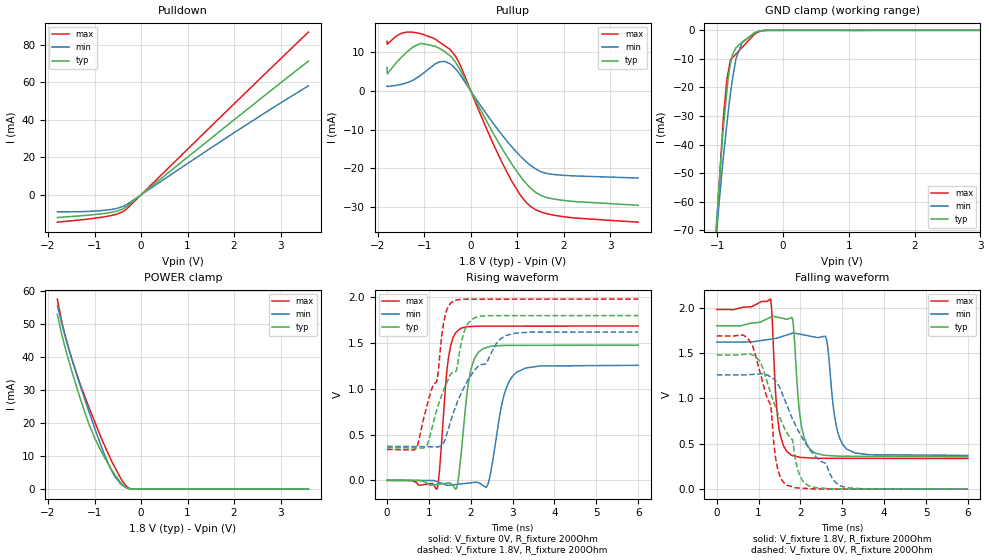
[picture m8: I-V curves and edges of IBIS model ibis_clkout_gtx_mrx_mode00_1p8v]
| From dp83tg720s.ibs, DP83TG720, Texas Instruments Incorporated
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| ibis_clkout_gtx_mrx_mode00_1p8v
[Model]   ibis_clkout_gtx_mrx_mode00_1p8v
Model_type   I/O
Polarity   Non-Inverting
Enable   Active-Low
Vinl = 0.54
Vinh = 1.26
Vmeas = 0.9
Vref = 0.9
Cref = 2pF
Rref = 100000
|   typ   min   max
C_comp   2.97pF   2.96pF   3.01pF
[Voltage Range]   1.8   1.62   1.98
[Temperature Range]   27   150   -40
[Pullup Reference]   1.8   1.62   1.98
[Pulldown Reference]   0   0   0
[Power Clamp Reference]   1.8   1.62   1.98
[GND Clamp Reference]   0   0   0
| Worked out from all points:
|   slope of the pulldown table from 0 to 0.27 V, typ, clamps not added: 49.7 ohm
|   slope of the pullup table from 0 to 0.27 V, typ, clamps not added: 43.2 ohm
|   GND clamp passes 1 mA (typ) near -0.44 V on its own axis
|   POWER clamp passes 1 mA (typ) near -0.37 V on its own axis
|   falling waveform, V_fixture 1.8V, R_fixture 200Ohm: 20-80 % time 172ps typ, 203ps min, 145ps max; typ from 1.8 V to 0.359 V
|   rising waveform, V_fixture 0V, R_fixture 200Ohm: 20-80 % time 219ps typ, 309ps min, 179ps max; typ from 0 V to 1.48 V
|   rising waveform, V_fixture 1.8V, R_fixture 200Ohm: 20-80 % time 662ps typ, 965ps min, 459ps max; typ from 0.359 V to 1.8 V
|   falling waveform, V_fixture 0V, R_fixture 200Ohm: 20-80 % time 691ps typ, 1.03ns min, 411ps max; typ from 1.48 V to 0 V
[Pulldown]
|   Voltage   I(typ)   I(min)   I(max)
-1.8V     -12.08mA   -9.033mA   -14.56mA
-1.125V   -10.8mA    -8.807mA   -12.86mA
-730.8mV  -9.674mA   -8.07mA    -11.45mA
-520.2mV  -8.646mA   -7.206mA   -10.24mA
-336.6mV  -6.645mA   -5.499mA   -8.007mA
2.072V    41.36mA    34.22mA    50.17mA
3.6V      71.25mA    58.08mA    86.69mA
[GND Clamp]
|   Voltage   I(typ)   I(min)   I(max)
-1.8V     -382.3mA   -332mA     -425.2mA
-1.017V   -68.67mA   -71.81mA   -70.53mA
-903.6mV  -32.69mA   -43.18mA   -29.12mA
-855mV    -21.28mA   -32.69mA   -17.07mA
-838.8mV  -17.47mA   -29.2mA    -15.06mA
-801mV    -11.68mA   -22.1mA    -10.37mA
-774mV    -8.705mA   -17.42mA   -9.699mA
-714.6mV  -6.046mA   -9.737mA   -8.229mA
-622.8mV  -4.089mA   -4.277mA   -5.956mA
-444.6mV  -1.097mA   -993.2uA   -1.545mA
-261mV    -16.1uA    -40.43uA   -15.49uA
3.6V      0A         0A         0A
[Pullup]
|   Voltage   I(typ)   I(min)   I(max)
-1.8V     6.066mA    1.271mA    12.85mA
-1.789V   4.411mA    1.14mA     12.09mA
-1.476V   8.918mA    1.762mA    15mA
-1.071V   12.31mA    4.113mA    14.83mA
-676.8mV  11.06mA    7.524mA    12.68mA
-444.6mV  9.086mA    7.025mA    10.74mA
-239.4mV  5.662mA    4.354mA    7.043mA
343.8mV   -7.902mA   -6.066mA   -9.904mA
797.4mV   -17.36mA   -13.27mA   -21.5mA
1.278V    -25.1mA    -19.23mA   -29.86mA
1.845V    -28.13mA   -21.74mA   -32.33mA
3.6V      -29.64mA   -22.58mA   -34.02mA
[POWER Clamp]
|   Voltage   I(typ)   I(min)   I(max)
-1.8V     53.01mA    55.74mA    57.65mA
-1.681V   45.61mA    49.02mA    49.43mA
-1.546V   38.55mA    42.1mA     42.27mA
-1.319V   27.98mA    31.92mA    32.33mA
-1.114V   19.49mA    23.28mA    24.54mA
-973.8mV  14.8mA     17.58mA    19.66mA
-666mV    6.684mA    6.531mA    9.544mA
-558mV    4.288mA    3.744mA    6.479mA
-444.6mV  2.137mA    1.736mA    3.468mA
-293.4mV  327.2uA    317.2uA    675uA
-109.8mV  6.037uA    13.6uA     2.646uA
3.6V      0A         0A         0A
[Ramp]
R_load = 200
|   typ   min   max
dV/dt_r   0.886179/2.19298e-10   0.754021/3.07889e-10   1.01172/1.7845e-10
dV/dt_f   0.864917/1.69904e-10   0.748861/2.02115e-10   0.985494/1.43915e-10
[Falling Waveform]
V_fixture = 1.8V
V_fixture_min = 1.62V
V_fixture_max = 1.98V
R_fixture = 200Ohm
C_fixture = 0F
|   Time   V(typ)   V(min)   V(max)
0s        1.8V       1.62V      1.98V
1.282ns   1.893V     1.652V     2.094V
1.469ns   1.892V     1.668V     730.9mV
1.761ns   1.885V     1.712V     380mV
2.029ns   683.2mV    1.704V     349.2mV
2.338ns   401.1mV    1.676V     341.9mV
2.622ns   371.7mV    1.65V      340.1mV
2.853ns   365.1mV    702mV      340mV
3.116ns   362.3mV    438.3mV    339.8mV
6ns       358.6mV    372mV      337.6mV
[Rising Waveform]
V_fixture = 0V
V_fixture_min = 0V
V_fixture_max = 0V
R_fixture = 200Ohm
C_fixture = 0F
|   Time   V(typ)   V(min)   V(max)
0s        1.712uV    26.55uV    886.7nV
1.194ns   -44.79mV   -13.6mV    -93.42mV
1.466ns   -28.61mV   -54.59mV   1.335V
1.746ns   185.5mV    -39.95mV   1.655V
1.983ns   1.165V     -27.56mV   1.68V
2.288ns   1.437V     -53.86mV   1.684V
2.457ns   1.462V     39.84mV    1.684V
2.811ns   1.474V     956mV      1.685V
3.095ns   1.474V     1.18V      1.685V
6ns       1.477V     1.257V     1.686V
[Rising Waveform]
V_fixture = 1.8V
V_fixture_min = 1.62V
V_fixture_max = 1.98V
R_fixture = 200Ohm
C_fixture = 0F
|   Time   V(typ)   V(min)   V(max)
0s        358.6mV    372mV      337.6mV
716.7ps   353.8mV    368.5mV    363.7mV
958.8ps   387.2mV    367.4mV    824.8mV
1.197ns   780.6mV    366.2mV    1.098V
1.305ns   929.9mV    385.4mV    1.571V
1.429ns   1.068V     506.8mV    1.864V
1.576ns   1.181V     724.1mV    1.957V
1.948ns   1.723V     1.105V     1.978V
2.838ns   1.799V     1.581V     1.979V
6ns       1.8V       1.62V      1.98V
[Falling Waveform]
|Gnd
V_fixture = 0V
V_fixture_min = 0V
V_fixture_max = 0V
R_fixture = 200Ohm
C_fixture = 0F
|   Time   V(typ)   V(min)   V(max)
0s        1.479V     1.259V     1.688V
837ps     1.482V     1.263V     1.597V
1.041ns   1.401V     1.27V      1.274V
1.285ns   1.059V     1.236V     930.4mV
1.375ns   942mV      1.209V     451.6mV
1.458ns   840.2mV    1.154V     218.6mV
1.67ns    626.8mV    929.7mV    45.07mV
2.059ns   87.21mV    551.6mV    9.743mV
2.954ns   3.257mV    37.15mV    2.567mV
6ns       1.733uV    26.43uV    649.9nV
